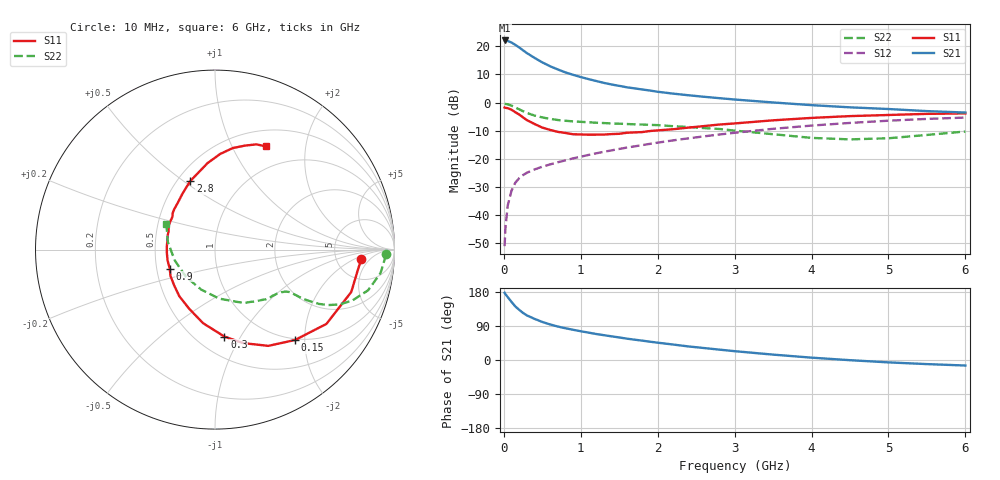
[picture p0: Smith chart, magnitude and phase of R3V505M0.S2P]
! SIEMENS Small Signal Semiconductors
! BFR181
! Si NPN RF Bipolar Junction Transistor in SOT23
! VCE = 0.5 V  IC = 5 mA
! Common Emitter S-Parameters:  May  1996
# GHz  S  MA  R  50
!  f  S11  S21  S12  S22
! GHz  MAG  ANG  MAG  ANG  MAG  ANG  MAG  ANG
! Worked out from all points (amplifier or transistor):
!   36 points, 10 MHz to 6 GHz, reference 50 ohm
!   highest |S21| = 22.1 dB at 10 MHz (marker M1)
!   |S21| within 3 dB of that: start of sweep to 224.8 MHz
!   unconditionally stable (mu >= 1): 587 MHz to end of sweep
!   at 250 MHz: K = 0.55, MSG = 22.2 dB, |S12| = -25.8 dB
!   at 1.4 GHz: K = 1.31, MAG = 8.4 dB, |S12| = -17.0 dB
!   at 6 GHz: K = 1.07, MAG = -0.7 dB, |S12| = -5.3 dB
!   S11 on the Smith chart (normalised r, x): 10 MHz: 9.13, -2.75; 150 MHz: 0.98, -1.80; 300 MHz: 0.67, -0.86; 900 MHz: 0.59, -0.13; 2.8 GHz: 0.58, +0.53; 6 GHz: 0.70, +1.37
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0.01  0.8177 -3.5  12.71 177.3  0.0028 92.6  0.9509 -1.6
0.02  0.8063 -7.1  12.63 174.0  0.0057 83.0  0.9465 -3.4
0.05  0.795 -17.3  12.46 166.0  0.0147 80.6  0.9315 -8.1
0.1  0.7462 -33.7  11.69 153.3  0.0272 72.2  0.8824 -14.9
0.15  0.6726 -48.5  10.6 141.1  0.0378 65.1  0.8154 -20.4
0.2  0.6132 -61.0  9.54 132.4  0.0453 61.0  0.7574 -23.8
0.25  0.5443 -73.2  8.487 124.1  0.0514 57.4  0.7027 -26.1
0.3  0.4875 -83.8  7.58 117.6  0.0566 55.9  0.6533 -27.6
0.4  0.4153 -99.2  6.222 108.5  0.0648 54.0  0.5873 -28.8
0.5  0.3595 -113.6  5.18 100.4  0.0724 53.5  0.5446 -29.3
0.6  0.327 -127.5  4.432 93.9  0.0795 54.0  0.5139 -29.4
0.7  0.302 -139.1  3.888 88.4  0.0867 54.7  0.4903 -29.6
0.9  0.2734 -157.2  3.117 79.7  0.1019 55.9  0.4637 -30.4
1.1  0.2687 -175.8  2.615 72.3  0.1172 56.8  0.447 -31.9
1.3  0.2699 169.7  2.24 65.5  0.1335 57.2  0.4327 -33.9
1.6  0.2908 152.4  1.867 56.3  0.1585 57.4  0.4159 -37.6
2.2  0.3357 127.5  1.443 40.8  0.2128 55.0  0.3804 -47.8
2.8  0.4065 109.7  1.198 27.4  0.2706 50.8  0.3394 -61.2
3.5  0.4837 94.9  1.005 14.2  0.3415 43.7  0.2739 -85.2
4.5  0.5748 80.0  0.823 -0.5  0.4348 31.4  0.2216 -137.1
5.5  0.6299 68.6  0.705 -10.8  0.5122 18.0  0.2657 171.1
6  0.6419 63.5  0.665 -14.6  0.5417 11.2  0.3062 152.3
